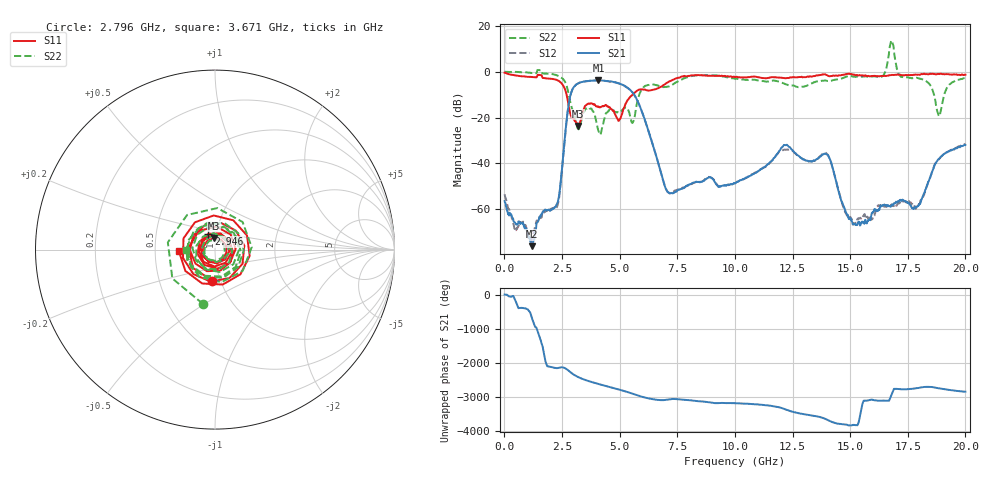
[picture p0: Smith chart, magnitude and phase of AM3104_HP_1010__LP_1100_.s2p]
!Created with skrf (http://scikit-rf.org).
# Hz S RI R 50.0
!freq ReS11 ImS11 ReS21 ImS21 ReS12 ImS12 ReS22 ImS22
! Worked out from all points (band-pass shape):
!   1601 points, 10 MHz to 20 GHz, reference 50 ohm
!   highest |S21| = -3.77 dB at 4.083 GHz (marker M1); lowest = -76.1 dB at 1.197 GHz (marker M2)
!   |S21| within 3 dB of the highest: 3.009 GHz to 5.308 GHz (2.299 GHz wide, 55.3 % of centre)
!   lowest |S11| = -23.7 dB at 3.183 GHz (marker M3), VSWR 1.14, Z = 49 + j6.39 ohm
!   |S11| at or under -10 dB: 2.697 GHz to 5.566 GHz (2.869 GHz wide, 69.4 % of centre)
!   |S22| runs from -27.5 to 13.6 dB; largest |S21 - S12| = 0.058
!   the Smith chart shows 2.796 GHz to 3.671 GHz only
!   S11 on the Smith chart (normalised r, x): 2.796 GHz: 0.92, -0.33; 2.946 GHz: 0.91, +0.16; 3.671 GHz: 0.66, -0.01
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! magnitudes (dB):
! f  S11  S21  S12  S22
! 10 MHz  -0.4  -56.4  -53.5  0.0
! 1.197 GHz  -2.3  -76.1  -72.8  -0.6
! 2.309 GHz  -3.8  -57.1  -58.4  -1.7
! 2.796 GHz  -15.2  -13.7  -13.8  -10.2
! 2.946 GHz  -20.4  -7.9  -7.9  -16.4
! 3.183 GHz  -23.7  -5.2  -5.2  -24.8
! 3.346 GHz  -20.1  -4.5  -4.6  -21.1
! 3.671 GHz  -13.9  -4.0  -4.1  -15.7
! 4.083 GHz  -15.2  -3.8  -3.8  -25.9
! 4.97 GHz  -21.3  -5.1  -5.1  -17.9
! 5.595 GHz  -9.6  -9.5  -9.6  -21.7
! 6.682 GHz  -7.2  -40.0  -40.1  -6.1
! 7.181 GHz  -4.1  -53.0  -53.1  -6.2
! 10.01 GHz  -2.4  -48.7  -48.7  -3.1
! 12.18 GHz  -2.8  -32.0  -34.1  -5.4
! 13.34 GHz  -2.1  -39.2  -39.2  -5.1
! 14.05 GHz  -1.8  -36.6  -36.7  -4.1
! 15.2 GHz  -1.4  -66.5  -66.4  -2.2
! 16.68 GHz  -1.6  -58.7  -58.0  7.3
! 17.93 GHz  -1.3  -58.8  -58.6  -2.8
! 18.85 GHz  -1.0  -38.0  -38.3  -19.4
! 20 GHz  -1.3  -32.0  -31.6  -2.8
